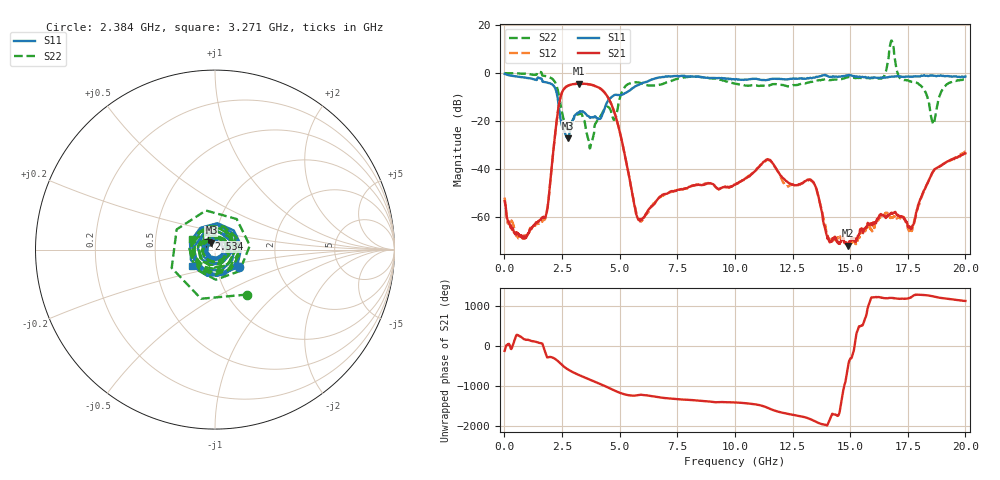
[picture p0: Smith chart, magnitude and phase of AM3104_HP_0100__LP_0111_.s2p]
!Created with skrf (http://scikit-rf.org).
# Hz S RI R 50.0
!freq ReS11 ImS11 ReS21 ImS21 ReS12 ImS12 ReS22 ImS22
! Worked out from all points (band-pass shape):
!   1601 points, 10 MHz to 20 GHz, reference 50 ohm
!   highest |S21| = -4.42 dB at 3.246 GHz (marker M1); lowest = -72.1 dB at 14.89 GHz (marker M2)
!   |S21| within 3 dB of the highest: 2.533 GHz to 4.28 GHz (1.748 GHz wide, 51.3 % of centre)
!   lowest |S11| = -27.3 dB at 2.746 GHz (marker M3), VSWR 1.09, Z = 47.9 + j3.67 ohm
!   |S11| at or under -10 dB: 2.303 GHz to 4.652 GHz (2.348 GHz wide, 67.5 % of centre)
!   |S22| runs from -31.5 to 13.6 dB; largest |S21 - S12| = 0.037
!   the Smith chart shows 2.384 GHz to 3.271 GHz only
!   S11 on the Smith chart (normalised r, x): 2.384 GHz: 1.28, -0.25; 2.534 GHz: 0.92, +0.11; 3.271 GHz: 0.76, -0.14
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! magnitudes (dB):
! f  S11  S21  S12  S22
! 10 MHz  -0.3  -53.5  -52.1  0.0
! 597.2 MHz  -1.5  -67.2  -68.4  -0.1
! 1.722 GHz  -3.7  -60.5  -61.3  -1.2
! 2.384 GHz  -15.6  -12.3  -12.4  -10.2
! 2.534 GHz  -23.1  -7.4  -7.4  -17.9
! 2.746 GHz  -27.3  -5.3  -5.3  -23.6
! 3.246 GHz  -16.5  -4.4  -4.5  -17.1
! 3.271 GHz  -16.1  -4.4  -4.5  -17.1
! 3.346 GHz  -16.0  -4.5  -4.5  -17.1
! 3.733 GHz  -18.7  -4.8  -4.8  -30.9
! 4.645 GHz  -10.0  -13.1  -13.2  -16.7
! 5.807 GHz  -5.0  -61.2  -61.1  -3.9
! 6.682 GHz  -1.9  -52.3  -52.5  -5.0
! 10.01 GHz  -2.7  -46.7  -46.7  -4.5
! 11.43 GHz  -2.8  -36.0  -36.2  -5.4
! 13.34 GHz  -2.1  -45.0  -45.2  -3.7
! 14.07 GHz  -1.5  -69.1  -69.6  -2.9
! 14.89 GHz  -0.9  -72.1  -72.1  -1.8
! 16.68 GHz  -1.6  -59.5  -59.6  7.2
! 17.64 GHz  -1.5  -65.3  -65.0  -3.6
! 18.6 GHz  -1.1  -41.1  -41.3  -21.3
! 20 GHz  -1.5  -33.6  -32.9  -2.5
